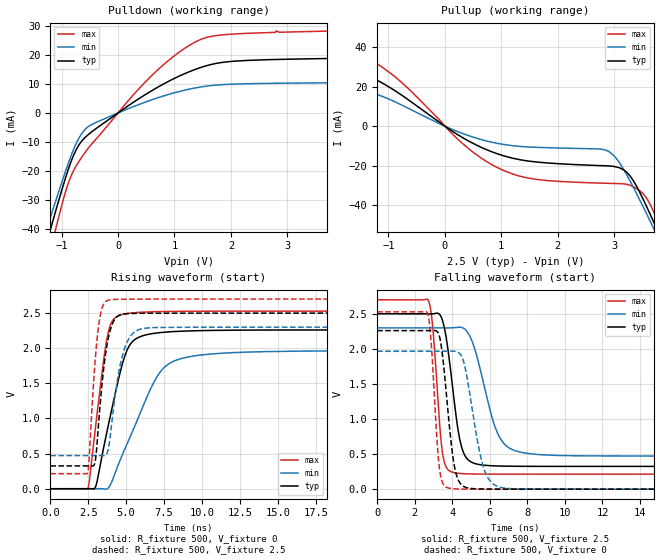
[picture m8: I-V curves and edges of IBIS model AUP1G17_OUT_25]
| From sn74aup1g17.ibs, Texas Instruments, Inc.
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[Model]   AUP1G17_OUT_25
Model_type  Output
Vref =   0
Rref =   1E6
Cref =   30p
Vmeas =   1.25
| variable   typ   min   max
C_comp   2.86pF   1.96pF   4.23pF
| C_pullup   3.21pF   1.96pF   4.23pF
| C_pulldown   2.51pF   2.22pF   3.08pF
[Temperature Range]   40   100   -40
| Ambient temperature   25   85   -40
[Voltage range]   2.5   2.3   2.7
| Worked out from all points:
|   slope of the pulldown table from 0 to 0.375 V, typ, clamps not added: 75.2 ohm
|   slope of the pullup table from 0 to 0.375 V, typ, clamps not added: 55.1 ohm
|   rising waveform, R_fixture 500, V_fixture 0: 20-80 % time 1.4ns typ, 2.4ns min, 861ps max; typ from 0 V to 2.26 V
|   falling waveform, R_fixture 500, V_fixture 2.5: 20-80 % time 633ps typ, 1.08ns min, 401ps max; typ from 2.5 V to 0.325 V
|   rising waveform, R_fixture 500, V_fixture 2.5: 20-80 % time 629ps typ, 807ps min, 485ps max; typ from 0.325 V to 2.5 V
|   falling waveform, R_fixture 500, V_fixture 0: 20-80 % time 517ps typ, 776ps min, 346ps max; typ from 2.26 V to 0 V
[Pulldown]
| AUP1G17_OUT_25
|   Voltage   I(typ)   I(min)   I(max)
-3.6V     -214mA     -193.5mA   -239.7mA
-1.26V    -44.55mA   -39.92mA   -52.42mA
-1.205V   -40.74mA   -36.52mA   -48.02mA
-1.115V   -34.57mA   -31.02mA   -40.91mA
-800mV    -15.22mA   -13.22mA   -20.4mA
-685mV    -10.84mA   -8.445mA   -16.54mA
-540mV    -7.689mA   -4.911mA   -12.5mA
675mV     8.558mA    5.038mA    14.35mA
1.105V    12.9mA     7.5mA      21.28mA
1.52V     16.03mA    9.129mA    25.76mA
2.585V    18.34mA    10.19mA    27.69mA
7.2V      19.61mA    10.73mA    29.61mA
[Pullup]
| AUP1G17_OUT_25
|   Voltage   I(typ)   I(min)   I(max)
-3.6V     37.28mA    23.5mA     50.35mA
-2.355V   24.65mA    15.21mA    35.57mA
-1.425V   26.01mA    17.2mA     35.58mA
-760mV    15.58mA    10.63mA    21.96mA
405mV     -7.279mA   -4.651mA   -11.04mA
1.05V     -15.07mA   -9.293mA   -22.54mA
2.845V    -20.04mA   -12.07mA   -28.88mA
3.17V     -22.17mA   -22.09mA   -29.2mA
3.455V    -33.67mA   -37.48mA   -32.73mA
3.685V    -47.61mA   -50.92mA   -42.5mA
3.82V     -56.28mA   -59.04mA   -51.47mA
7.2V      -294.7mA   -278.7mA   -311.5mA
[Ramp]
| AUP1G17_OUT_25
| variable   typ   min   max
dV/dt_r   1.36/1.40E-09   1.18/2.40E-09   1.52/8.62E-10
dV/dt_f   1.31/6.39E-10   1.10/1.09E-09   1.50/4.08E-10
R_load = 500
[Rising Waveform]
| AUP1G17_OUT_25
R_fixture =   500
C_fixture =   0
L_fixture =   0
V_fixture =   0
V_fixture_min = 0
V_fixture_max = 0
|   Time   V(typ)   V(min)   V(max)
0s        19.04nV    76.96nV    1.464nV
2.48ns    345.3uV    -28.45uV   8.697mV
3.01ns    43.89mV    514.5uV    932mV
3.73ns    809.4mV    -2.332mV   2.132V
4.045ns   1.126V     95.54mV    2.372V
4.58ns    1.636V     395.6mV    2.469V
5.615ns   2.13V      917.2mV    2.507V
7.185ns   2.221V     1.646V     2.521V
8.715ns   2.243V     1.858V     2.526V
32.79ns   2.261V     1.966V     2.528V
[Falling Waveform]
| AUP1G17_OUT_25
R_fixture =   500
C_fixture =   0
L_fixture =   0
V_fixture =   2.5
V_fixture_min = 2.3
V_fixture_max = 2.7
|   Time   V(typ)   V(min)   V(max)
0s        2.5V       2.3V       2.7V
2.735ns   2.5V       2.3V       2.685V
2.965ns   2.501V     2.3V       2.299V
3.475ns   2.409V     2.3V       528.6mV
4.035ns   1.413V     2.301V     239.5mV
4.4ns     710mV      2.309V     224mV
4.795ns   432.2mV    2.245V     218.2mV
6.395ns   330.7mV    808.4mV    214.5mV
7.58ns    326.1mV    531.2mV    214.4mV
32.79ns   324.7mV    472mV      214.4mV
[Rising Waveform]
| AUP1G17_OUT_25
R_fixture =   500
C_fixture =   0
L_fixture =   0
V_fixture =   2.5
V_fixture_min = 2.3
V_fixture_max = 2.7
|   Time   V(typ)   V(min)   V(max)
0s        324.7mV    472mV      214.4mV
2.46ns    325mV      472mV      224.5mV
2.94ns    366.9mV    472.2mV    1.779V
3.125ns   767.6mV    472mV      2.217V
3.405ns   1.482V     471mV      2.568V
3.77ns    2.087V     522.3mV    2.681V
4.17ns    2.384V     1.157V     2.694V
4.74ns    2.483V     1.885V     2.698V
5.93ns    2.497V     2.272V     2.699V
32.79ns   2.5V       2.3V       2.7V
[Falling Waveform]
| AUP1G17_OUT_25
R_fixture =   500
C_fixture =   0
L_fixture =   0
V_fixture =   0
V_fixture_min = 0
V_fixture_max = 0
|   Time   V(typ)   V(min)   V(max)
0s        2.261V     1.966V     2.528V
2.69ns    2.261V     1.966V     2.505V
2.87ns    2.261V     1.966V     2.113V
3.305ns   2.189V     1.966V     323.7mV
3.765ns   1.13V      1.967V     18.99mV
4.075ns   388.6mV    1.967V     6.234mV
4.4ns     91.21mV    1.933V     2.243mV
5.645ns   1.758mV    327.8mV    78.48uV
6.565ns   262.7uV    26.05mV    13.15uV
32.79ns   -69.36nV   4.241nV    -41.47nV
